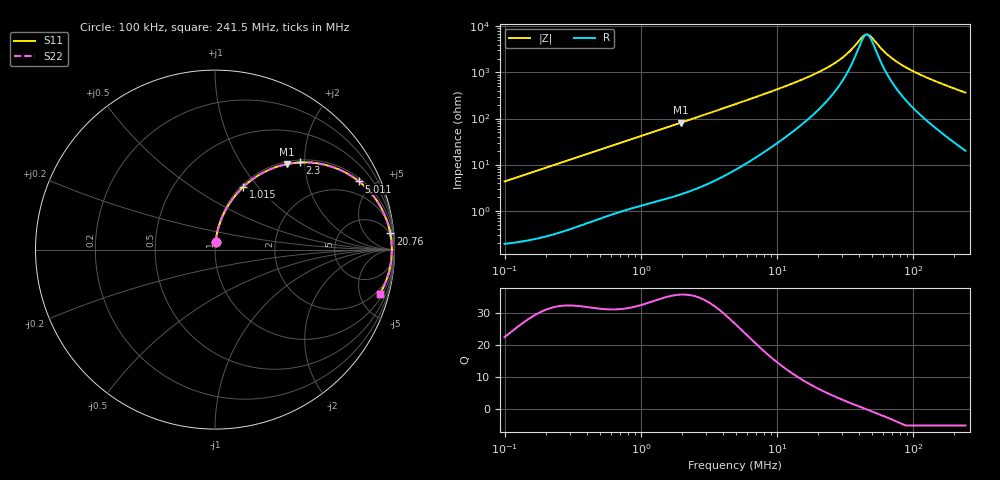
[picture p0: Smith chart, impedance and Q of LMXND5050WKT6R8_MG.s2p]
! LMXND5050WKT6R8_MG  S-PARAMETER MODEL  ( General Type )
! Model Generated by TAIYO YUDEN Corporation (http://www.ty-top.com)
! Version 1.0
! TAIYO YUDEN Control No. 191023NI43SB-FBB
! Copyright(c) 2019 TAIYO YUDEN CO.,LTD. All Rights Reserved.
! Product Description (link to TY-COMPAS)
! https://ds.yuden.co.jp/TYCOMPAS/or/detail?pn=LMXND5050WKT6R8MMG&u=M
! Products Name : Inductors
! Characteristics :
!  Inductance : 6.8 uH , SRF(min) : 30 MHz , DC Resistance(max) : 0.108 Ohm
!  Rated Current : Saturation :1600 mA , Temp Rise : 1650 mA
!  Case Size : 4.9 x 4.9 / 0.193 x 0.193 [mm/inch] , Thickness : 2 / 0.079 [mm/inch]
!  (Conditions: Temperature = 25 degC , DC Bias Current/Voltage = 0A / 0V)
! External Node Assignments :
!  1  o---GGG---o  2
! GND o---------o GND
! Frequency Range : 0.1MHz  -  241.513628MHz  [ 402 STEP ]
# MHz S RI R 50
! Freq[MHz].  S11 Real  S11 Imag  S21 Real  S21 Imag  S12 Real  S12 Imag  S22 Real  S22 Imag
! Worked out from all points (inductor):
!   401 points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, 100 kHz to 241.5 MHz, reference 50 ohm
!   read as one part in series: L = 6.81 uH near 104 kHz
!   highest Q = 35.9 at 1.968 MHz (marker M1), where L = 6.55 uH
!   self-resonance near 45.6 MHz
!   S11 on the Smith chart (normalised r, x): 100 kHz: 1.00, +0.09; 1.015 MHz: 1.03, +0.84; 2.3 MHz: 1.05, +1.89; 5.011 MHz: 1.16, +4.15; 20.76 MHz: 4, +21; 241.5 MHz: 1.40, -7.29
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0.1  0.00372 0.0427  0.9963 -0.0427  0.9963 -0.0427  0.00372 0.0427
0.368674  0.0283 0.151  0.9717 -0.151  0.9717 -0.151  0.0283 0.151
0.648494  0.0757 0.2489  0.9243 -0.2489  0.9243 -0.2489  0.0757 0.2489
1.014904  0.1583 0.35  0.8417 -0.35  0.8417 -0.35  0.1583 0.35
1.359207  0.2462 0.4165  0.7538 -0.4165  0.7538 -0.4165  0.2462 0.4165
1.967774  0.3993 0.476  0.6007 -0.476  0.6007 -0.476  0.3993 0.476
2.299503  0.4735 0.4855  0.5265 -0.4855  0.5265 -0.4855  0.4735 0.4855
3.264874  0.6401 0.4651  0.3599 -0.4651  0.3599 -0.4651  0.6401 0.4651
4.914404  0.7968 0.3841  0.2032 -0.3841  0.2032 -0.3841  0.7968 0.3841
5.011044  0.8028 0.3794  0.1972 -0.3794  0.1972 -0.3794  0.8028 0.3794
8.644385  0.9182 0.2462  0.0818 -0.2462  0.0818 -0.2462  0.9182 0.2462
18.11814  0.9729 0.1088  0.0271 -0.1088  0.0271 -0.1088  0.9729 0.1088
20.76419  0.9769 0.0897  0.0231 -0.0897  0.0231 -0.0897  0.9769 0.0897
30.65223  0.9834 0.0423  0.0166 -0.0423  0.0166 -0.0423  0.9834 0.0423
35.12882  0.9845 0.0274  0.0155 -0.0274  0.0155 -0.0274  0.9845 0.0274
41.85813  0.9852 0.00891  0.0148 -0.00891  0.0148 -0.00891  0.9852 0.00891
45.24902  0.9853 0.000802  0.0147 -0.000802  0.0147 -0.000802  0.9853 0.000802
48.91461  0.9852 -0.00731  0.0148 0.00731  0.0148 0.00731  0.9852 -0.00731
66.79689  0.9836 -0.0406  0.0164 0.0406  0.0164 0.0406  0.9836 -0.0406
82.75365  0.9809 -0.0654  0.0191 0.0654  0.0191 0.0654  0.9809 -0.0654
108.6901  0.9748 -0.1011  0.0252 0.1011  0.0252 0.1011  0.9748 -0.1011
241.5136  0.9185 -0.2476  0.0815 0.2476  0.0815 0.2476  0.9185 -0.2476
